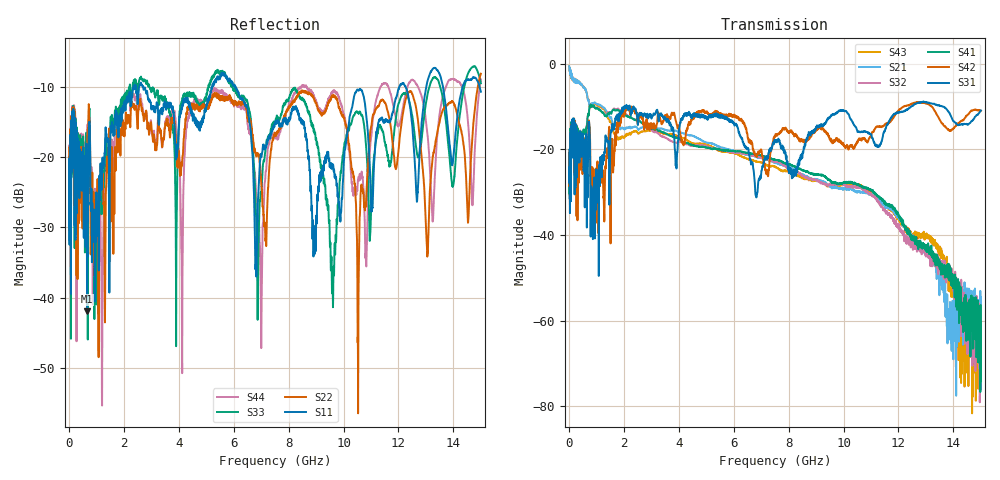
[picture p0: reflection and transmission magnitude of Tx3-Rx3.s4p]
! FILE: N:\QM 2007\Prüfprotokolle\Highspeed\Konfektionierte Ltg\L45593-D106\D30\8216\0002  kpl\IL  mit Chris Boards\Tx3-Rx3.s4p
# MHz S DB R 50.00
! FREQ  S11  S12  S13  S14
!  S21  S22  S23  S24
!  S31  S32  S33  S34
!  S41  S42  S43  S44
!  DB  ANG  DB  ANG  DB  ANG  DB  ANG
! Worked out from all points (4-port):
!   2999 points, 10 MHz to 15 GHz, reference 50 ohm
!   strongest paths, dB at 10 MHz, 3.755 GHz, 7.505 GHz, 11.26 GHz, 15 GHz:
!     S31: -24.3, -14.9, -18.2, -19.4, -10.9
!     S42: -25.1, -11.4, -17.1, -14.6, -11.0
!     S41: -30.3, -17.0, -22.4, -30.9, -64.4
!     S32: -29.4, -18.1, -22.8, -32.3, -76.1
!     S21: -0.6, -15.6, -23.1, -31.3, -55.1
!     S43: -0.6, -16.5, -24.0, -31.5, -64.7
!   lowest |S11| = -42.0 dB at 665 MHz (marker M1), VSWR 1.02, Z = 49.2 + j0.0504 ohm
!   |S11| at or under -10 dB: start of sweep to 2.359 GHz; 2.703 GHz to 5.22 GHz (2.517 GHz wide, 63.5 % of centre); 6.071 GHz to 12.03 GHz (5.962 GHz wide, 65.9 % of centre)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
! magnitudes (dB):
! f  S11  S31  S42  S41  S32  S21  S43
! 10 MHz  -21.1  -24.3  -25.1  -30.3  -29.4  -0.6  -0.6
! 665 MHz  -42.0  -25.8  -17.4  -13.9  -13.3  -7.5  -7.4
! 7 GHz  -19.9  -25.9  -20.1  -21.4  -21.9  -22.0  -23.0
! 8.22 GHz  -13.1  -25.2  -16.5  -24.0  -25.0  -24.6  -25.9
! 9.6 GHz  -21.4  -12.0  -18.4  -27.6  -28.2  -28.8  -28.3
! 10.77 GHz  -12.1  -15.7  -17.5  -28.9  -29.4  -30.1  -29.0
! 15 GHz  -10.7  -10.9  -11.0  -64.4  -76.1  -55.1  -64.7
